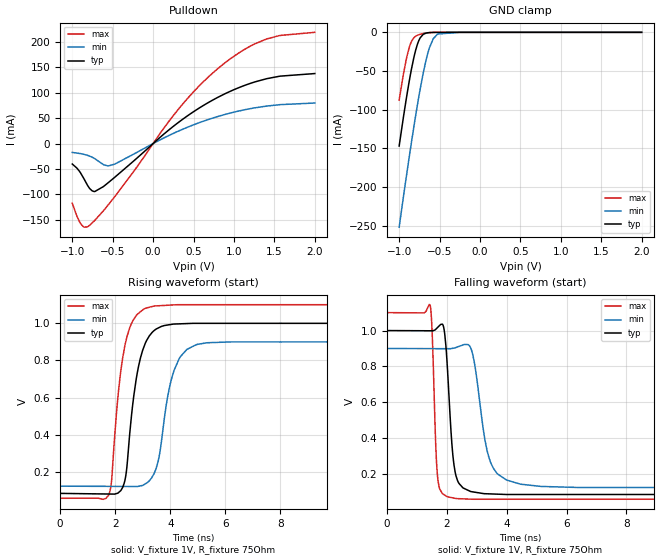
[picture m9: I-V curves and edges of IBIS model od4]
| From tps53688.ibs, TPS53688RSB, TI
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|   od4 Model
[Model]   od4
Model_type   Open_drain
Polarity   Non-Inverting
Vmeas = 0.5
Vref = 1
Cref = 2pF
Rref = 75
|   typ   min   max
C_comp   2.803pF   2.739pF   2.895pF
[Voltage Range]   1   0.9   1.1
|Junction Temperature
[Temperature Range]   25   125   -40
[Pullup Reference]   1   0.9   1.1
[Pulldown Reference]   0   0   -0
[Power Clamp Reference]   1   0.9   1.1
[GND Clamp Reference]   0   0   0
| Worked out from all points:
|   slope of the pulldown table from 0 to 0.15 V, typ, clamps not added: 7.18 ohm
|   GND clamp passes 1 mA (typ) near -0.67 V on its own axis
|   falling waveform, V_fixture 1V, R_fixture 75Ohm: 20-80 % time 217ps typ, 443ps min, 124ps max; typ from 1 V to 0.086 V
|   rising waveform, V_fixture 1V, R_fixture 75Ohm: 20-80 % time 475ps typ, 546ps min, 449ps max; typ from 0.086 V to 1 V
[Pulldown]
|   Voltage   I(typ)   I(min)   I(max)
-1V       -40.23mA   -17.47mA   -117.3mA
-910mV    -54.78mA   -19.42mA   -154mA
-856mV    -69.06mA   -21.17mA   -164.4mA
-784mV    -88.51mA   -24.74mA   -160.5mA
-721mV    -94.27mA   -29.73mA   -150.9mA
-559mV    -77.41mA   -44.06mA   -121.3mA
-475mV    -66.31mA   -40.43mA   -104.5mA
296mV     39.51mA    23.31mA    64.2mA
794mV     90.34mA    52.9mA     146.5mA
1.094V    112.1mA    65.21mA    181.6mA
1.406V    127.6mA    73.79mA    205.8mA
2V        137.7mA    79.76mA    218.8mA
[GND Clamp]
|   Voltage   I(typ)   I(min)   I(max)
-1V       -146.9mA   -251.7mA   -87.47mA
-916mV    -88.68mA   -189.9mA   -37.03mA
-874mV    -62.43mA   -160.2mA   -19.23mA
-820mV    -33.52mA   -123.3mA   -7.234mA
-772mV    -14.86mA   -92.52mA   -3.761mA
-739mV    -6.999mA   -72.78mA   -2.534mA
-703mV    -2.685mA   -53.06mA   -1.567mA
-631mV    -399.4uA   -21.84mA   -442.3uA
-577mV    -105.6uA   -8.071mA   -129.8uA
-523mV    -27.84uA   -2.198mA   -31.95uA
-250mV    0A         -974.2nA   0A
2V        0A         0A         0A
[POWER Clamp]
|   Voltage   I(typ)   I(min)   I(max)
-1V       0A         0A         0A
2V        0A         0A         0A
[Ramp]
R_load = 75
|   typ   min   max
dV/dt_r   0.54854/4.74847e-10   0.465317/5.45561e-10   0.624273/4.49612e-10
dV/dt_f   0.54854/2.1566e-10   0.465317/4.4066e-10   0.624273/1.2426e-10
[Falling Waveform]
V_fixture = 1V
V_fixture_min = 0.9V
V_fixture_max = 1.1V
R_fixture = 75Ohm
C_fixture = 0F
|   Time   V(typ)   V(min)   V(max)
0s        1V         900mV      1.1V
1.438ns   998.8mV    899.3mV    1.144V
1.669ns   1.014V     899.2mV    226mV
1.871ns   1.031V     899.1mV    89.39mV
2.272ns   215.2mV    903.7mV    65.22mV
2.857ns   101.4mV    871.7mV    60.01mV
3.336ns   90.5mV     337.5mV    60.01mV
3.644ns   88.64mV    210.8mV    60.01mV
6.406ns   86.51mV    125.5mV    60mV
500ns     85.77mV    124.5mV    59.54mV
[Rising Waveform]
V_fixture = 1V
V_fixture_min = 0.9V
V_fixture_max = 1.1V
R_fixture = 75Ohm
C_fixture = 0F
|   Time   V(typ)   V(min)   V(max)
0s        85.77mV    124.5mV    59.54mV
1.765ns   82.37mV    123.5mV    78.37mV
2.272ns   118.4mV    123.2mV    814.3mV
2.79ns    724.1mV    122.9mV    1.046V
3.228ns   928.9mV    151.7mV    1.085V
3.558ns   973.6mV    257.9mV    1.093V
3.963ns   991.3mV    649.8mV    1.096V
4.261ns   995.7mV    788.5mV    1.099V
6.2ns     998.9mV    899.1mV    1.099V
500ns     1V         900mV      1.1V
